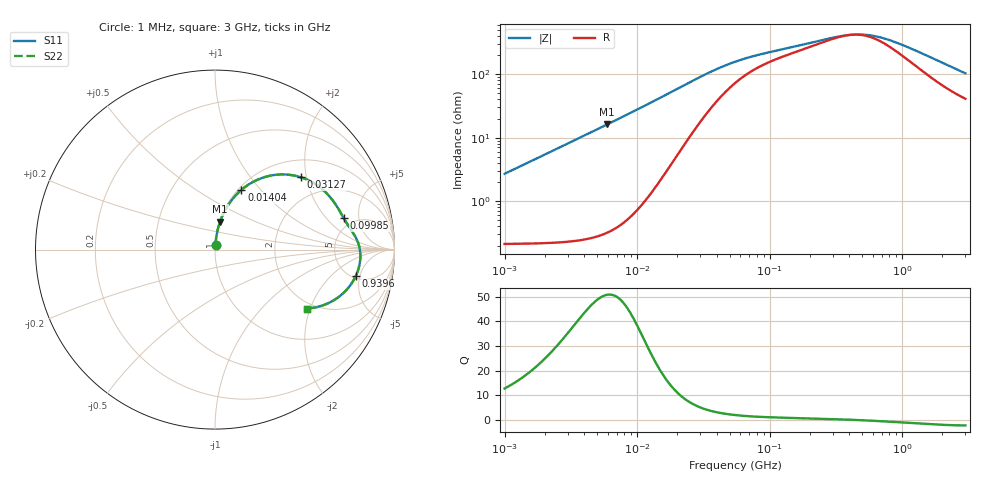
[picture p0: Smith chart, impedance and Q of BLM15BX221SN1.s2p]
! BLM15BX221SN1
# Hz S RI R 50
!Freq.(Hz) S11(Real) S11(Imag) S21(Real) S21(Imag) S12(Real) S12(Imag) S22(Real) S22(Imag)
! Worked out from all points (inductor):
!   401 points, 1 MHz to 3 GHz, reference 50 ohm
!   read as one part in series: L = 428 nH near 1.041 MHz
!   highest Q = 50.8 at 5.938 MHz (marker M1), where L = 433 nH
!   self-resonance near 415.8 MHz
!   S11 on the Smith chart (normalised r, x): 1 MHz: 1.00, +0.05; 14.04 MHz: 1.04, +0.79; 31.27 MHz: 1.40, +1.85; 99.85 MHz: 4.12, +3.17; 939.6 MHz: 5.31, -4.32; 3 GHz: 1.82, -1.89
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1000000  0.00283 0.0268  0.9972 -0.0268  0.9972 -0.0268  0.00283 0.0268
2097170  0.00534 0.0561  0.9947 -0.0561  0.9947 -0.0561  0.00534 0.0561
3823119  0.0129 0.1017  0.9871 -0.1017  0.9871 -0.1017  0.0129 0.1017
5938264  0.0283 0.1564  0.9717 -0.1564  0.9717 -0.1564  0.0283 0.1564
9600343  0.0711 0.2448  0.9289 -0.2448  0.9289 -0.2448  0.0711 0.2448
1.404268e7  0.1473 0.3329  0.8527 -0.3329  0.8527 -0.3329  0.1473 0.3329
1.461624e7  0.1586 0.3422  0.8414 -0.3422  0.8414 -0.3422  0.1586 0.3422
2.225279e7  0.3203 0.4142  0.6797 -0.4142  0.6797 -0.4142  0.3203 0.4142
3.127247e7  0.4778 0.4031  0.5222 -0.4031  0.5222 -0.4031  0.4778 0.4031
4.138676e7  0.5817 0.3492  0.4183 -0.3492  0.4183 -0.3492  0.5817 0.3492
5.477226e7  0.6486 0.2836  0.3514 -0.2836  0.3514 -0.2836  0.6486 0.2836
9.984923e7  0.7174 0.1748  0.2826 -0.1748  0.2826 -0.1748  0.7174 0.1748
2.094008e8  0.771 0.0906  0.229 -0.0906  0.229 -0.0906  0.771 0.0906
3.318279e8  0.7988 0.0332  0.2012 -0.0332  0.2012 -0.0332  0.7988 0.0332
4.480278e8  0.8086 -0.0118  0.1914 0.0118  0.1914 0.0118  0.8086 -0.0118
5.929311e8  0.8088 -0.0592  0.1912 0.0592  0.1912 0.0592  0.8088 -0.0592
8.005644e8  0.7969 -0.1155  0.2031 0.1155  0.2031 0.1155  0.7969 -0.1155
9.395906e8  0.7842 -0.1476  0.2158 0.1476  0.2158 0.1476  0.7842 -0.1476
1.243477e9  0.7487 -0.2055  0.2513 0.2055  0.2513 0.2055  0.7487 -0.2055
1.613037e9  0.6977 -0.2571  0.3023 0.2571  0.3023 0.2571  0.6977 -0.2571
2.266846e9  0.6041 -0.3096  0.3959 0.3096  0.3959 0.3096  0.6041 -0.3096
3e9  0.5111 -0.3282  0.4889 0.3282  0.4889 0.3282  0.5111 -0.3282
